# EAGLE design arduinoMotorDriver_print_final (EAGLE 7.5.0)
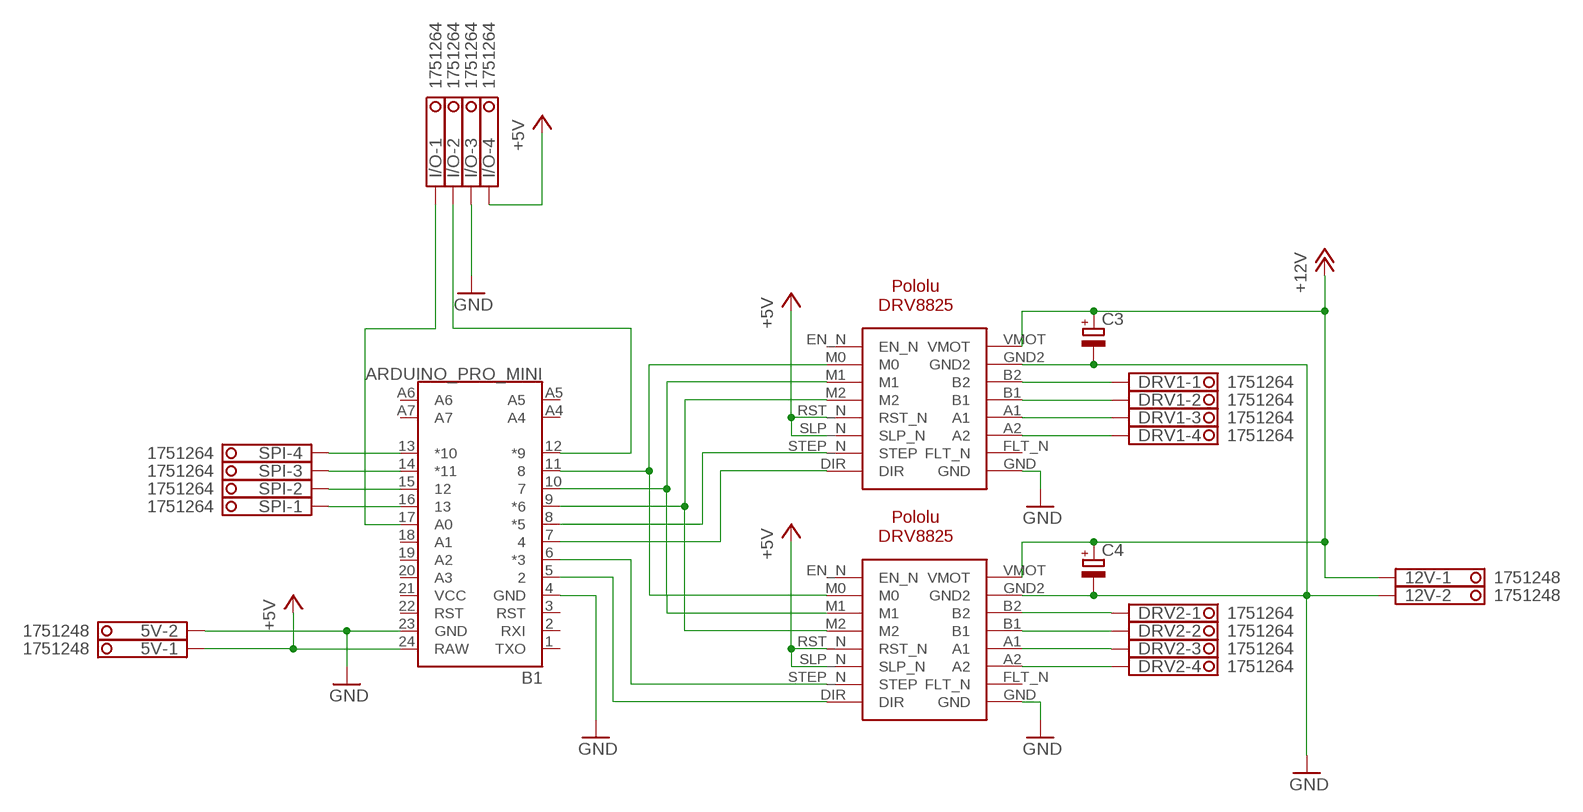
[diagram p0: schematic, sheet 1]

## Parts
5V  1751248  [1751248]
12V  1751248  [1751248]
B1  ARDUINO_PRO_MINI  [ARDUINO_PRO_MINI]
C3  CPOL-EUE3.5-10  [E3,5-10]
C4  CPOL-EUE3.5-10  [E3,5-10]
DRV1  1751264  [1751264]
DRV2  1751264  [1751264]
I/O  1751264  [1751264]
SPI  1751264  [1751264]
U$4  POLOLU-DRV8825  [POLOLU-DRV8825]
U$5  POLOLU-DRV8825  [POLOLU-DRV8825]

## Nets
+5V: 5V.1 B1.24(RAW) I/O.4 U$4.RST_N U$4.SLP_N U$5.RST_N U$5.SLP_N
+12V: 12V.1 C3.+ C4.+ U$4.VMOT U$5.VMOT
GND: 5V.2 12V.2 B1.4(GND) B1.23(GND) C3.- C4.- I/O.3 U$4.GND U$4.GND2 U$5.GND U$5.GND2
N$1: B1.11 U$4.M0 U$5.M0
N$2: B1.10 U$4.M1
N$3: B1.9(*6) U$4.M2 U$5.M2
N$4: B1.13(*10) SPI.4
N$5: B1.8(*5) U$4.STEP_N(STEP)
N$6: B1.7 U$4.DIR
N$7: U$5.M1
N$8: B1.14(*11) SPI.3
N$9: B1.6(*3) U$5.STEP_N(STEP)
N$10: B1.5 U$5.DIR
N$11: DRV1.4 U$4.A2
N$12: DRV1.3 U$4.A1
N$13: DRV1.2 U$4.B1
N$14: DRV1.1 U$4.B2
N$15: DRV2.4 U$5.A2
N$16: DRV2.3 U$5.A1
N$17: DRV2.2 U$5.B1
N$18: DRV2.1 U$5.B2
N$19: B1.15 SPI.2
N$20: B1.17(A0) I/O.1
N$21: B1.12(*9) I/O.2
N$22: B1.16 SPI.1
Unconnected: B1.1(TXO) B1.2(RXI) B1.3(RST) B1.18(A1) B1.19(A2) B1.20(A3) B1.22(RST) B1.A4 B1.A5 B1.A6 B1.A7 U$4.EN_N U$4.FLT_N U$5.EN_N U$5.FLT_N

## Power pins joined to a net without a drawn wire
VCC: B1.21(VCC)

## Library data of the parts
5V 12V = con-phoenix-350:1751248: MKDS 1/ 2-3,5 Printklemme; OC_FARNELL: unknown; OC_NEWARK: unknown
B1 = SparkFun-Boards:ARDUINO_PRO_MINI: SparkFun Pro Mini Pro Mini compatible footprint. Dimensions: 0.7 x 1.3" PCB Thickness: 0.8mm SparkFun Products: 3.3V/8MHz 5V/16MHz
C3 C4 = rcl:CPOL-EU: POLARIZED CAPACITOR, European symbol
DRV1 DRV2 I/O SPI = con-phoenix-350:1751264: MKDS 1/ 4-3,5 Printklemme Nennstrom: 10 A Bemessungsspannung: 160 V Raster: 3,5 mm Polzahl: 4 Montageart: Löten Anschlussart: Schraubanschluss Anschlussrichtung vom Leiter zur Platine: 0° Source: http://eshop.phoenixcontact.com .. 1751264.pdf; MPN: 1751264; OC_FARNELL: unknown; OC_NEWARK: 10R0934
U$4 U$5 = eae:POLOLU-DRV8825

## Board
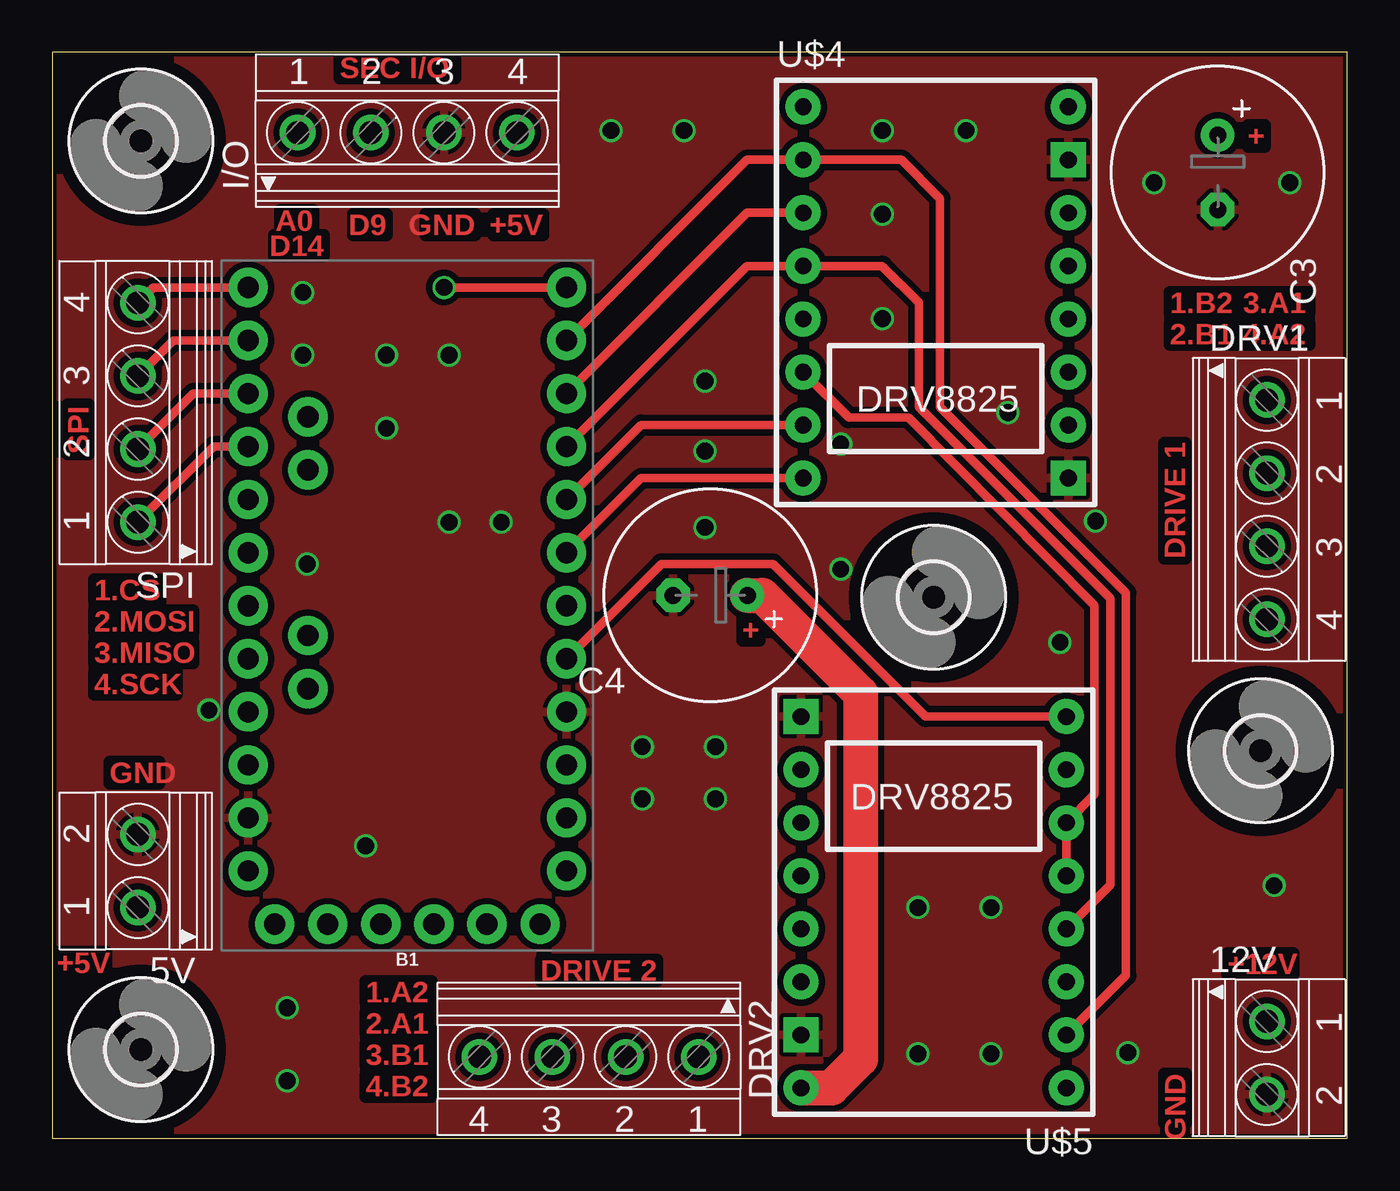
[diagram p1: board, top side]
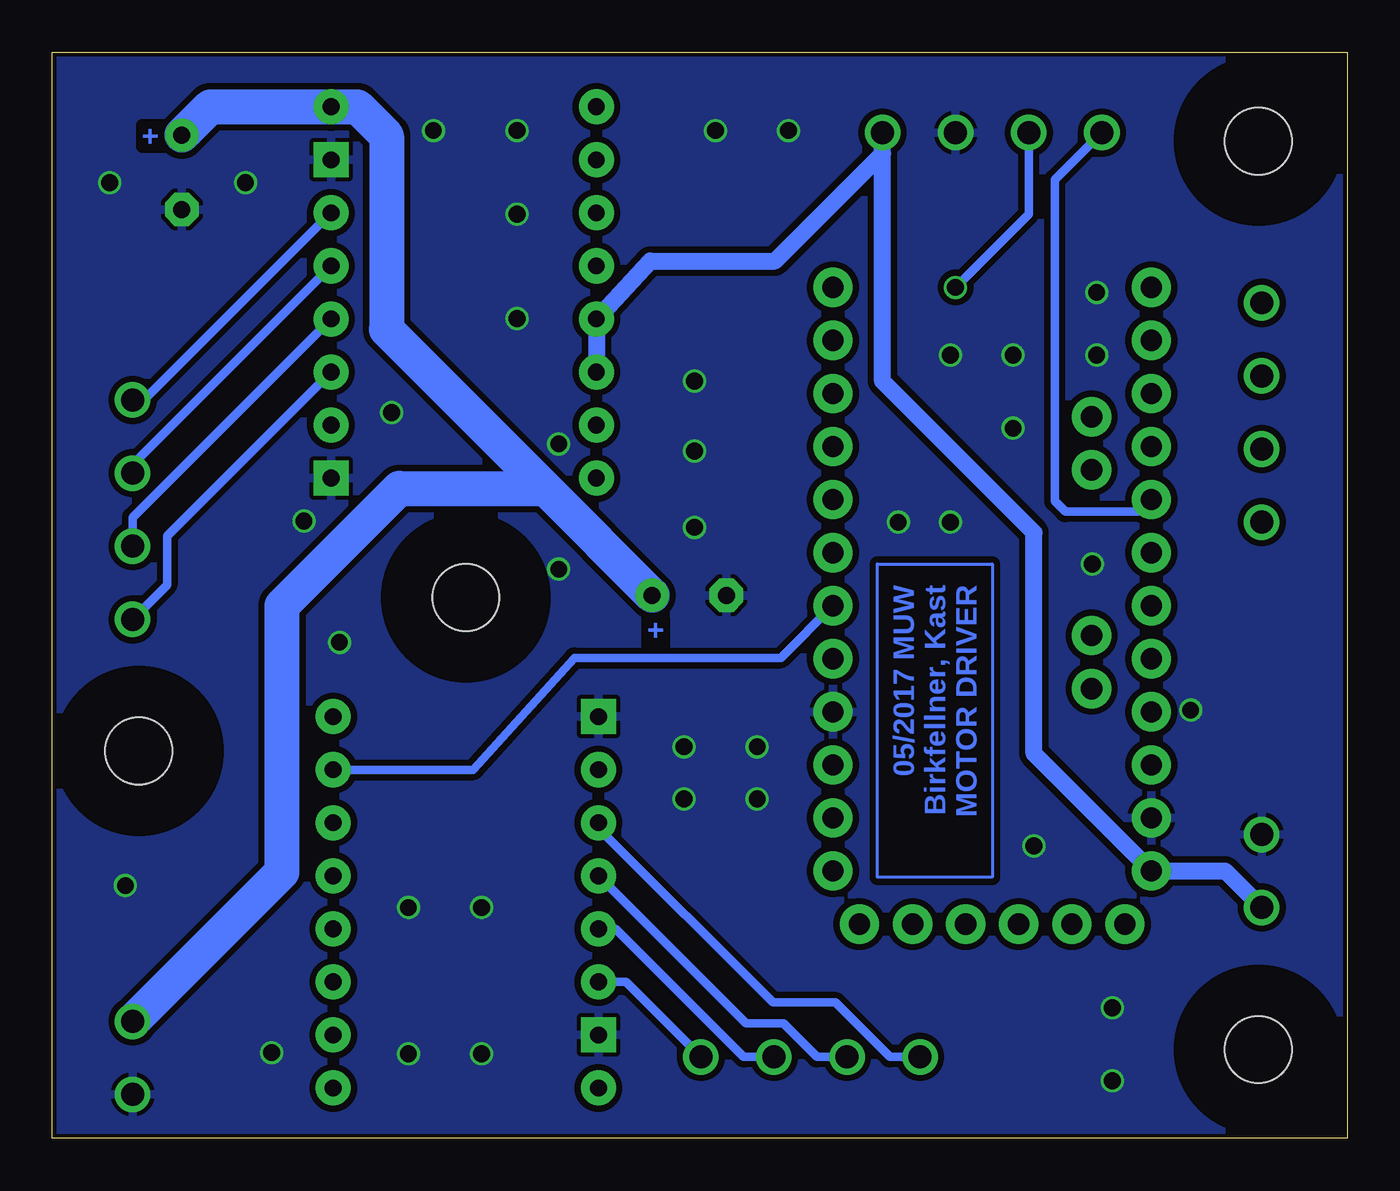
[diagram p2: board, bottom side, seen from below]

Size 62 x 52 mm. Coordinates in mm from the lower left corner, seen from the top.
Outline: 0,0 62,0 62,52 0,52 0,0
Copper layers (1*16): Top 0.035mm / dielectric 1.5mm / Bottom 0.035mm
Design rules "Eagle-DRU - 1506 - LeitOn - 01 and 02 layers - STANDARD *": minimum track width 0.15mm, minimum drill 0.3mm, track to track 0.3mm, track to pad 0.3mm, pad to pad 0.3mm, via to via 0.3mm, smd to smd 0.3mm, copper to edge 0.2mm, drill to drill 0.25mm, minimum pad ring 0.15mm, minimum via ring 0.15mm, stop-mask expansion 0.05mm, vias tented up to drill 0mil, thermal gap 0.2mm

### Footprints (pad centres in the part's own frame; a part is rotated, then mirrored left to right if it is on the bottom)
1751248 = drill 1.1 pad 1.7: 1 -1.75,-0.1; 2 1.75,-0.1
ARDUINO_PRO_MINI = drill 1.016 pad 1.88: 1 -7.62,12.7; 2 -7.62,10.16; 3 -7.62,7.62; 4 -7.62,5.08; 5 -7.62,2.54; 6 -7.62,0; 7 -7.62,-2.54; 8 -7.62,-5.08; 9 -7.62,-7.62; 10 -7.62,-10.16; 11 -7.62,-12.7; 12 -7.62,-15.24; 13 7.62,-15.24; 14 7.62,-12.7; 15 7.62,-10.16; 16 7.62,-7.62; 17 7.62,-5.08; 18 7.62,-2.54; 19 7.62,0; 20 7.62,2.54; 21 7.62,5.08; 22 7.62,7.62; 23 7.62,10.16; 24 7.62,12.7; A4 4.763,1.429; A5 4.763,3.969; A6 4.763,-9.049; A7 4.763,-6.509; BLK -6.35,15.24; GND -3.81,15.24; GRN 6.35,15.24; RXI 1.27,15.24; TXO 3.81,15.24; VCC -1.27,15.24
E3,5-10 = drill 0.813 pad 1.6: + -1.778,0 | drill 0.813 pad 1.6 octagon: - 1.778,0
1751264 = drill 1.1 pad 1.7: 1 -5.25,-0.1; 2 -1.75,-0.1; 3 1.75,-0.1; 4 5.25,-0.1
3,2 = hole 3.2: 0,0
POLOLU-DRV8825 = drill 0.8 pad 1.676: A1 6.35,-1.27; A2 6.35,-3.81; B1 6.35,1.27; B2 6.35,3.81; DIR -6.35,-8.89; EN_N -6.35,8.89; FLT_N 6.35,-6.35; M0 -6.35,6.35; M1 -6.35,3.81; M2 -6.35,1.27; RST_N -6.35,-1.27; SLP_N -6.35,-3.81; STEP_N -6.35,-6.35; VMOT 6.35,8.89 | drill 0.8 pad 1.676 square: GND 6.35,-8.89; GND2 6.35,6.35

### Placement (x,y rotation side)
5V  4,12.8 90 top
12V  58.25,3.85 270 top
B1  17,25.5 180 top
C3  55.8,46.25 270 top
C4  31.5,26 180 top
DRV1  58.25,30.1 270 top
DRV2  25.7,3.8 180 top
I/O  17,48.25 0 top
SPI  4,34.75 90 top
U$1  [3,2]  42.2,25.9 0 top
U$2  [3,2]  4.25,47.75 0 top
U$3  [3,2]  57.85,18.55 0 top
U$4  42.3,40.5 0 top
U$5  42.2,11.3 180 top
U$6  [3,2]  4.25,4.25 0 top

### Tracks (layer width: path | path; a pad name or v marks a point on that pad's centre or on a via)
+5V
  Top 0.406: U$4.SLP_N 38.14,34.5 41,34.5 49.9,25.5 49.9,16.46 U$5.SLP_N U$5.RST_N
  Bottom 0.813: U$4.SLP_N U$4.RST_N 33.38,42 27.4,42 22.25,47.15 I/O.4 22.25,36.25 15,29 15,18.42 B1.24 5.85,12.8 5V.1
+12V
  Top 1.676: U$5.VMOT 37.31,2.41 38.7,3.8 38.7,21.3 34,26 C4.+
  Bottom 1.676: 12V.1 51,12.75 51,25.5 45.39,31.11 38.39,31.11 | C3.+ 54.44,49.39 U$4.VMOT 47.39,49.39 46,48 46,38.72 38.39,31.11 | 38.39,31.11 C4.+
GND  (via drill 0.8)
  other vias: 28.25,18.75 31.75,18.75 31.75,16.25 28.25,16.25 26.75,48.25 30.25,48.25 39.75,44.25 39.75,39.25 31.25,32.9 37.75,27.25 48.25,23.75 39.75,48.25 43.75,48.25 15,14 19,37.5 7.5,20.5 44.95,11.05 41.45,11.05 41.45,4.05 44.95,4.05 58.5,12.1 51.5,4.1 52.75,45.75 59.25,45.75 31.25,29.25 31.25,36.25 37.75,33.25 49.95,29.55 45.75,34.75 11.25,6.25 11.25,2.75 12,37.5 12,40.5 16,37.5 16,34 19,29.5 21.5,29.5 12.2,27.5
  pour Bottom: 0,52 62,52 62,0 0,0
  pour Top: 0,52 62,52 62,0 0,0
N$1
  Top 0.406: B1.11 33.27,46.85 U$4.M0 40.65,46.85 42.5,45 42.5,35 51.4,26.1 51.4,7.8 U$5.M0
N$2
  Top 0.406: B1.10 33.27,44.31 U$4.M1
N$3
  Top 0.406: B1.9 33.27,41.77 U$4.M2 39.73,41.77 41.5,40 41.5,35 50.65,25.85 50.65,12.13 U$5.M2
N$4
  Top 0.406: B1.13 4.84,40.74 SPI.4
N$5
  Top 0.406: B1.8 28.19,34.15 U$4.STEP_N
N$6
  Top 0.406: B1.7 28.19,31.61 U$4.DIR
N$8
  Top 0.406: B1.14 5.8,38.2 SPI.3
N$9
  Bottom 0.406: U$5.STEP_N 41.85,17.65 37,23 27.12,23 B1.6
N$10
  Top 0.406: U$5.DIR 41.81,20.19 34.5,27.5 29.16,27.5 B1.5
N$11
  Bottom 0.406: U$4.A2 56.5,28.84 56.5,26.5 DRV1.4
N$12
  Bottom 0.406: U$4.A1 58.15,29.73 DRV1.3
N$13
  Bottom 0.406: U$4.B1 58.15,32.27 DRV1.2
N$14
  Bottom 0.406: U$4.B2 57.61,35.35 DRV1.1
N$15
  Bottom 0.406: DRV2.4 21.9,3.9 24.5,6.5 27.5,6.5 35.85,14.85 U$5.A2
N$16
  Bottom 0.406: DRV2.3 25.4,3.9 27,5.5 28.78,5.5 U$5.A1
N$17
  Bottom 0.406: DRV2.2 28.9,3.9 35.03,10.03 U$5.B1
N$18
  Bottom 0.406: DRV2.1 34.54,7.49 U$5.B2
N$19
  Top 0.406: B1.15 6.76,35.66 SPI.2
N$20
  Bottom 0.406: B1.17 9.96,30 13.5,30 14,30.5 14,45.9 I/O.1
N$21  (via drill 0.8)
  Top 0.406: B1.12 v18.76,40.74
  Bottom 0.406: I/O.2 15.25,44.25 v18.76,40.74
N$22
  Top 0.406: B1.16 7.72,33.12 SPI.1
N$60
  Bottom 0.152: 17,27.5 17,12.5 22.5,12.5 22.5,27.5 17,27.5

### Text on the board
Top: SEC I/O | + | A0 | D9 | GND | +5V | D14 | 1.B2 | 3.A1 | 2.B1 | 4.A2 | SPI | DRIVE 1 | 1.CS | + | 2.MOSI | 3.MISO | 4.SCK | GND | DRIVE 2 | +5V | +12V | 1.A2 | 2.A1 | 3.B1 | GND | 4.B2
Bottom: + | MOTOR DRIVER | Birkfellner, Kast | 05/2017 MUW | +

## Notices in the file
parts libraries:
SparkFun-Boards: Licensing: Creative Commons ShareAlike 4.0 International - https://creativecommons.org/licenses/by-sa/4.0
